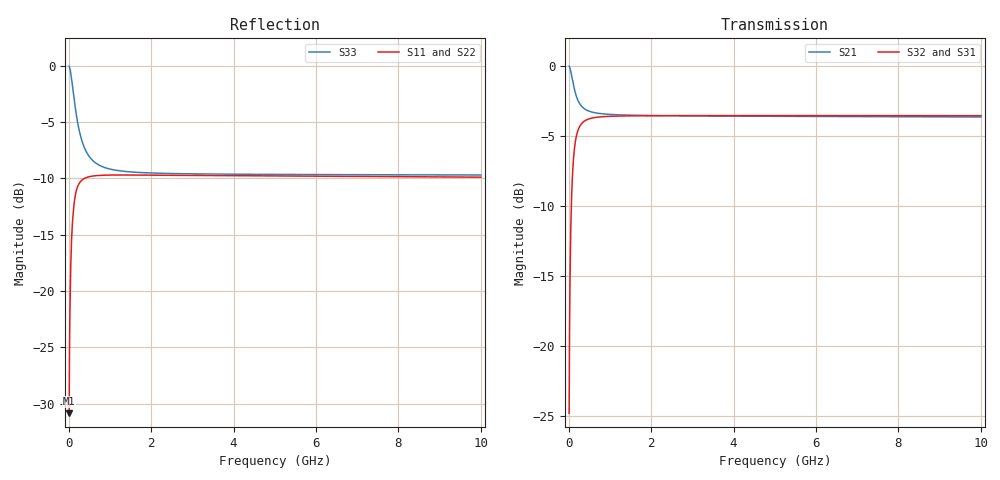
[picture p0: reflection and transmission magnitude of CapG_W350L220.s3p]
! Created Fri Sep 09 14:38:02 2011
# ghz S ma R 50
! 3 Port Network Data from SP1.SP block
! freq  magS11  angS11  magS12  angS12  magS13  angS13
!  magS21  angS21
!  magS22  angS22  magS23  angS23
!  magS31  angS31  magS32  angS32
!  magS33  angS33
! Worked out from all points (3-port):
!   1000 points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, 10 MHz to 10 GHz, reference 50 ohm
!   strongest paths, dB at 10 MHz, 2.51 GHz, 5.01 GHz, 7.51 GHz, 10 GHz:
!     S32: -24.8, -3.6, -3.6, -3.6, -3.6
!     S31: -24.8, -3.6, -3.6, -3.6, -3.6
!     S21: 0.0, -3.6, -3.6, -3.6, -3.7
!   lowest |S11| = -30.9 dB at 10 MHz (marker M1), VSWR 1.06, Z = 49.7 - j2.84 ohm
!   |S11| at or under -10 dB: start of sweep to 379.4 MHz
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0.01  0.02865 -94.7  0.9978 -1.6  0.05732 85.1
      0.9978 -1.6  0.02865 -94.7  0.05732 85.1
      0.05732 85.1  0.05732 85.1  0.9967 -6.6
0.08  0.186 -124.1  0.908 -9.8  0.3725 55.8
      0.908 -9.8  0.186 -124.1  0.3726 55.8
      0.3725 55.8  0.3726 55.8  0.847 -46.7
0.14  0.2521 -140.5  0.8236 -11.7  0.5076 40.2
      0.8236 -11.7  0.2521 -140.4  0.5076 40.2
      0.5076 40.2  0.5076 40.2  0.6926 -71.1
0.2  0.2855 -149.6  0.7682 -11.1  0.5723 30.6
     0.7682 -11.1  0.2855 -149.6  0.5723 30.7
     0.5723 30.6  0.5723 30.7  0.5838 -88.5
0.27  0.3036 -156.6  0.7314 -9.8  0.6091 23.7
      0.7314 -9.8  0.3036 -156.6  0.6091 23.7
      0.6091 23.7  0.6091 23.7  0.5029 -103.3
0.52  0.3227 -167.6  0.6868 -6.2  0.6485 12.8
      0.6868 -6.2  0.3227 -167.6  0.6485 12.8
      0.6485 12.8  0.6485 12.8  0.391 -132.6
0.94  0.3273 -173.5  0.6719 -3.8  0.6599 7.1
      0.6719 -3.8  0.3273 -173.4  0.6599 7.2
      0.6599 7.1  0.6599 7.2  0.3504 -152.0
1.65  0.3274 -176.8  0.6658 -2.4  0.6633 4.0
      0.6658 -2.4  0.3274 -176.7  0.6633 4.1
      0.6633 4.0  0.6633 4.1  0.3366 -163.8
5.01  0.3244 -180.0  0.6605 -1.2  0.6642 1.2
      0.6605 -1.2  0.3245 -179.9  0.6643 1.2
      0.6642 1.2  0.6643 1.2  0.3295 -175.0
10  0.3204 178.6  0.6568 -1.2  0.6637 0.5
    0.6568 -1.2  0.3205 178.7  0.6638 0.5
    0.6637 0.5  0.6638 0.5  0.3276 -178.0
